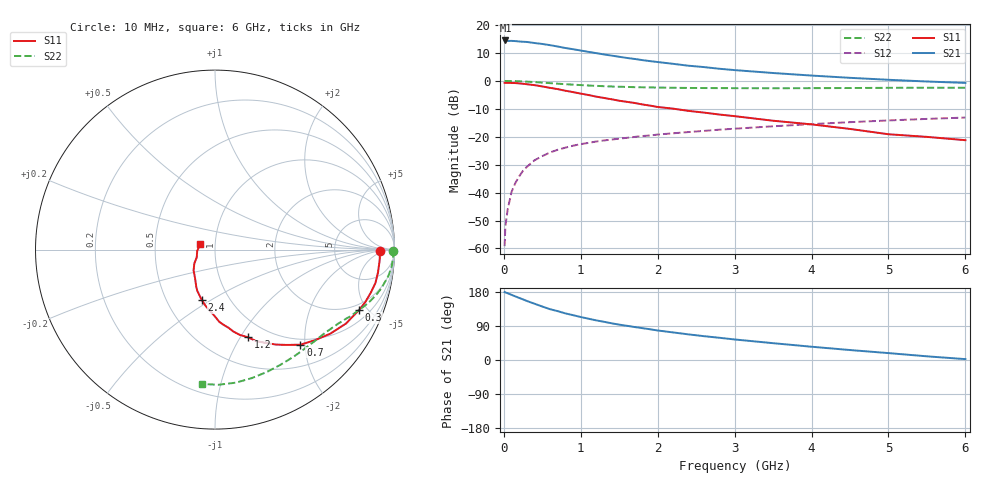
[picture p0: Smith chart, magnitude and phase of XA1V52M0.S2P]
! SIEMENS Discrete & RF Semiconductors
! BFY180
! Si NPN RF Bipolar Junction Transistor in MICRO-X
! VCE = 1.5 V  IC = 2 mA
! Common Emitter S-Parameters:  May  1997
# GHz  S  MA  R  50
!  f  S11  S21  S12  S22
! GHz  MAG  ANG  MAG  ANG  MAG  ANG  MAG  ANG
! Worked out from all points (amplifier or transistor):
!   36 points, 10 MHz to 6 GHz, reference 50 ohm
!   highest |S21| = 14.5 dB at 20 MHz (marker M1)
!   |S21| within 3 dB of that: start of sweep to 869.3 MHz
!   unconditionally stable (mu >= 1): 2.179 GHz to end of sweep
!   at 250 MHz: K = 0.16, MSG = 23.1 dB, |S12| = -32.1 dB
!   at 1.4 GHz: K = 0.79, MSG = 15.0 dB, |S12| = -21.0 dB
!   at 6 GHz: K = 1.12, MAG = 4.1 dB, |S12| = -13.1 dB
!   S11 on the Smith chart (normalised r, x): 10 MHz: 24, -3; 300 MHz: 1.60, -4.43; 700 MHz: 0.89, -1.91; 1.2 GHz: 0.80, -1.08; 2.4 GHz: 0.74, -0.46; 6 GHz: 0.85, +0.05
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0.01  0.921 -0.6  5.19 179.4  0.0011 83.3  0.9938 -0.3
0.02  0.919 -1.7  5.286 178.2  0.0025 92.1  0.9959 -0.8
0.05  0.9194 -3.7  5.172 176.1  0.005 84.2  0.994 -1.7
0.1  0.917 -7.9  5.194 172.0  0.0103 86.0  0.9913 -3.6
0.2  0.9011 -15.3  5.067 163.8  0.0196 80.4  0.9827 -7.0
0.3  0.8705 -22.7  4.968 155.7  0.029 76.0  0.9674 -10.2
0.5  0.7944 -36.2  4.574 141.1  0.045 68.0  0.9312 -15.9
0.6  0.7508 -42.3  4.356 134.1  0.0523 64.8  0.9104 -18.4
0.7  0.7118 -48.1  4.121 128.9  0.0584 61.3  0.8909 -20.6
0.8  0.666 -52.9  3.872 123.0  0.0638 59.2  0.8717 -22.6
1.1  0.5578 -65.9  3.3 109.0  0.0776 53.3  0.8261 -27.7
1.2  0.522 -69.4  3.138 104.6  0.0821 51.6  0.814 -29.4
1.5  0.4411 -80.3  2.699 93.3  0.0925 48.2  0.7849 -33.7
1.7  0.4023 -86.7  2.468 87.0  0.0992 46.5  0.7711 -36.4
2  0.3409 -95.1  2.173 77.9  0.1094 44.2  0.7591 -40.5
2.2  0.3182 -99.4  2.018 72.8  0.1152 42.6  0.7523 -43.3
2.4  0.2902 -104.8  1.867 67.6  0.1213 41.4  0.7469 -45.9
3  0.2335 -116.4  1.558 54.2  0.1392 37.3  0.7401 -53.8
3.5  0.1934 -125.2  1.382 44.4  0.1538 34.0  0.7382 -60.4
4.5  0.1379 -146.5  1.133 26.3  0.1823 26.7  0.7446 -74.0
5.5  0.0994 -176.1  0.974 9.7  0.2085 18.8  0.7532 -88.4
6  0.0867 159.3  0.919 2.3  0.2205 14.4  0.7528 -95.7
